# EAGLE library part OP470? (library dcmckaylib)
Low-noise quad op-amp 5nV/Hz^(0.5) voltage noise 6MHz bandwidth Low Offset voltage drift 2uV/C 1.7pA/Hz^(0.5) @ 10Hz, 0.4pA/Hz^(0.4) @1kHz current noise
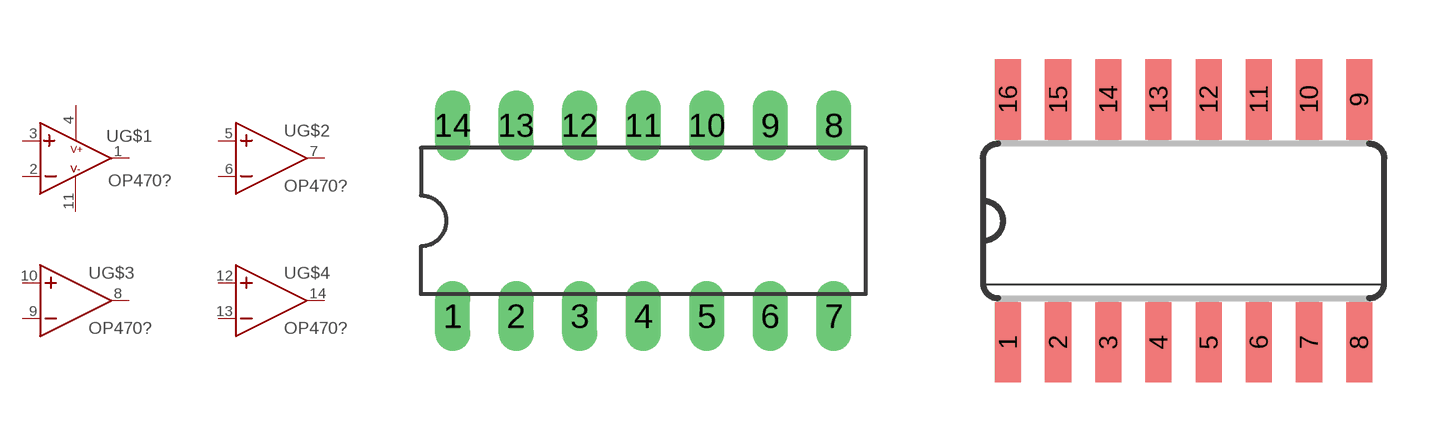
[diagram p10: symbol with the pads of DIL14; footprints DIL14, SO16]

Designator prefix U; gates G$1=OPAMP2 G$2=OPAMP G$3=OPAMP G$4=OPAMP

## OP470P  [DIL14]
1  G$1:OUT  out
2  G$1:IN-  in
3  G$1:IN+  in
4  G$1:V+  pwr
5  G$2:IN+  in
6  G$2:IN-  in
7  G$2:OUT  out
8  G$3:OUT  out
9  G$3:IN-  in
10  G$3:IN+  in
11  G$1:V-  pwr
12  G$4:IN+  in
13  G$4:IN-  in
14  G$4:OUT  out

## OP470S  [SO16]
1  G$1:OUT  out
2  G$1:IN-  in
3  G$1:IN+  in
4  G$1:V+  pwr
5  G$2:IN+  in
6  G$2:IN-  in
7  G$2:OUT  out
10  G$3:OUT  out
11  G$3:IN-  in
12  G$3:IN+  in
13  G$1:V-  pwr
14  G$4:IN+  in
15  G$4:IN-  in
16  G$4:OUT  out

## Footprint DIL14 (pad centres in mm)
Dual In Line Package
drill 0.889 long: 1 -7.62,-3.81; 2 -5.08,-3.81; 3 -2.54,-3.81; 4 0,-3.81; 5 2.54,-3.81; 6 5.08,-3.81; 7 7.62,-3.81; 8 7.62,3.81; 9 5.08,3.81; 10 2.54,3.81; 11 0,3.81; 12 -2.54,3.81; 13 -5.08,3.81; 14 -7.62,3.81

## Footprint SO16 (pad centres in mm)
Small Outline package 150 mil
smd 0.66 x 2.032: 1 -4.445,-3.073; 2 -3.175,-3.073; 3 -1.905,-3.073; 4 -0.635,-3.073; 5 0.635,-3.073; 6 1.905,-3.073; 7 3.175,-3.073; 8 4.445,-3.073; 9 4.445,3.073; 10 3.175,3.073; 11 1.905,3.073; 12 0.635,3.073; 13 -0.635,3.073; 14 -1.905,3.073; 15 -3.175,3.073; 16 -4.445,3.073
